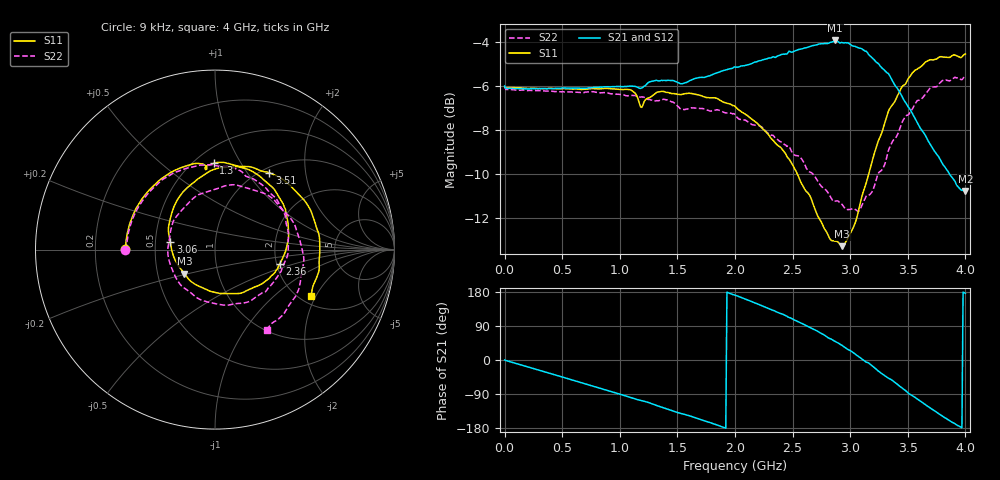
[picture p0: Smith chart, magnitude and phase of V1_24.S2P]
! ZVRE, 3.40
! symbol freq-unit parameter-type data-format keyword impedance-ohm
#  HZ  S  RI  R  50
! freq  reS11  imS11  reS21  imS21  reS12  imS12  reS22  imS22
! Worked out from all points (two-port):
!   401 points, 9 kHz to 4 GHz, reference 50 ohm
!   highest |S21| = -3.91 dB at 2.87 GHz (marker M1); lowest = -10.8 dB at 4 GHz (marker M2)
!   |S21| within 3 dB of the highest: start of sweep to 3.5 GHz
!   lowest |S11| = -13.3 dB at 2.93 GHz (marker M3), VSWR 1.55, Z = 34.3 - j9.62 ohm
!   |S11| at or under -10 dB: 2.541 GHz to 3.161 GHz (619.1 MHz wide, 21.7 % of centre)
!   |S22| runs from -11.7 to -5.5 dB; largest |S21 - S12| = 0.024
!   S11 on the Smith chart (normalised r, x): 9 kHz: 0.33, +0.00; 1.3 GHz: 0.62, +0.77; 2.36 GHz: 2.09, -0.37; 3.06 GHz: 0.60, +0.06; 3.51 GHz: 1.08, +1.28; 4 GHz: 2.28, -1.83
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9000  -0.5 0.00153  0.5019 0.000832  0.5024 -0.00113  -0.5004 -0.000608
3.200083e8  -0.4595 0.1851  0.4344 -0.2383  0.4389 -0.2362  -0.4528 0.1871
6.700075e8  -0.3429 0.354  0.2457 -0.4307  0.252 -0.4296  -0.3301 0.3554
9.600068e8  -0.1943 0.4544  0.0312 -0.4995  0.0351 -0.5028  -0.1838 0.4447
1.300006e9  -0.00624 0.4806  -0.2412 -0.4562  -0.2381 -0.4603  0.0297 0.4629
1.340006e9  0.0262 0.4862  -0.2726 -0.4376  -0.272 -0.4428  0.054 0.4618
1.640005e9  0.2179 0.4297  -0.4536 -0.2559  -0.4523 -0.2608  0.2244 0.3872
2.000004e9  0.393 0.2216  -0.5481 0.087  -0.5501 0.0807  0.3962 0.173
2.200004e9  0.4076 0.0524  -0.4819 0.308  -0.4875 0.3031  0.4081 -0.00913
2.360004e9  0.3615 -0.0775  -0.3525 0.4676  -0.3638 0.4622  0.3515 -0.1455
2.530003e9  0.2558 -0.1938  -0.1436 0.5877  -0.1565 0.5892  0.2199 -0.2703
2.670003e9  0.1227 -0.2451  0.0768 0.6155  0.0674 0.6217  0.0699 -0.3098
2.870003e9  -0.1146 -0.1906  0.4197 0.48  0.4109 0.4879  -0.1671 -0.2176
2.930002e9  -0.1706 -0.1335  0.4939 0.3923  0.5035 0.3894  -0.2146 -0.1632
3.060002e9  -0.2491 0.0441  0.6022 0.1264  0.6074 0.1284  -0.2593 0.0292
3.190002e9  -0.2214 0.2548  0.5625 -0.1511  0.5691 -0.1465  -0.1803 0.2248
3.340001e9  -0.0124 0.4445  0.3469 -0.4031  0.3528 -0.4041  0.0641 0.3569
3.450001e9  0.1915 0.462  0.1348 -0.4558  0.1406 -0.4638  0.2692 0.3149
3.510001e9  0.303 0.4283  0.00896 -0.4476  0.0268 -0.4575  0.3641 0.2344
3.710001e9  0.5427 0.1928  -0.2326 -0.2797  -0.2362 -0.286  0.4944 -0.0702
3.82e9  0.584 0.0127  -0.291 -0.1535  -0.2948 -0.1539  0.4524 -0.2544
4e9  0.5348 -0.2589  -0.2887 0.0205  -0.2879 0.0244  0.2874 -0.4455
